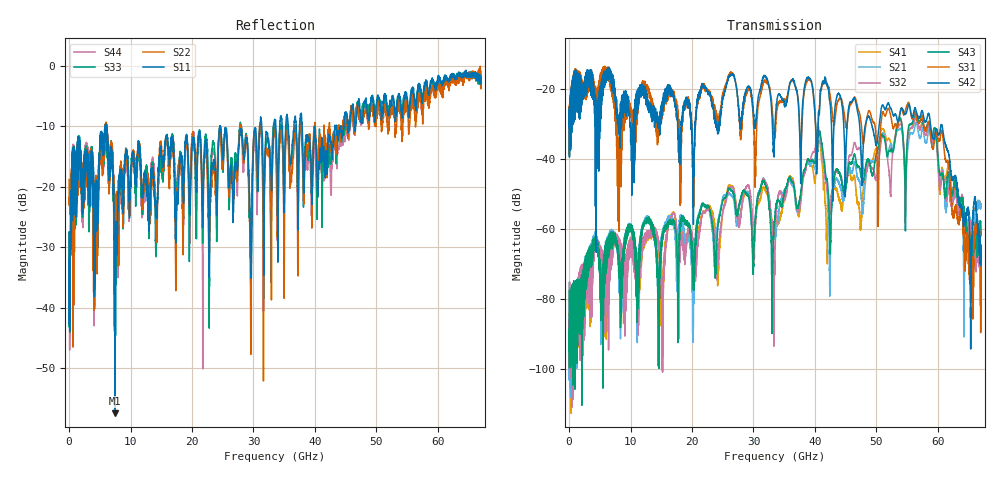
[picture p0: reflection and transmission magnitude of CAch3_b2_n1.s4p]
!Agilent Technologies,N5247A,US51170199,A.09.90.13
!Agilent N5247A: A.09.90.13
!Date: Wednesday, October 17, 2018 17:19:54
!Correction: S11(Full 4 Port(1,2,3,4))
!S12(Full 4 Port(1,2,3,4))
!S13(Full 4 Port(1,2,3,4))
!S14(Full 4 Port(1,2,3,4))
!S21(Full 4 Port(1,2,3,4))
!S22(Full 4 Port(1,2,3,4))
!S23(Full 4 Port(1,2,3,4))
!S24(Full 4 Port(1,2,3,4))
!S31(Full 4 Port(1,2,3,4))
!S32(Full 4 Port(1,2,3,4))
!S33(Full 4 Port(1,2,3,4))
!S34(Full 4 Port(1,2,3,4))
!S41(Full 4 Port(1,2,3,4))
!S42(Full 4 Port(1,2,3,4))
!S43(Full 4 Port(1,2,3,4))
!S44(Full 4 Port(1,2,3,4))
!S4P File: Measurements: <S11,S12,S13,S14>,
!<S21,S22,S23,S24>,
!<S31,S32,S33,S34>,
!<S41,S42,S43,S44>:
# Hz S  dB  R 50
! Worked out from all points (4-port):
!   6701 points, 10 MHz to 67 GHz, reference 50 ohm
!   strongest paths, dB at 10 MHz, 16.76 GHz, 33.51 GHz, 50.25 GHz, 67 GHz:
!     S42: -31.1, -20.4, -30.1, -33.6, -68.2
!     S31: -30.3, -21.1, -33.2, -50.9, -83.5
!     S43: -90.9, -57.6, -56.7, -37.1, -57.9
!     S32: -98.4, -56.1, -64.7, -42.6, -75.1
!     S21: -93.8, -56.8, -68.0, -39.7, -53.5
!     S41: -84.3, -55.7, -61.0, -37.0, -53.4
!   lowest |S11| = -57.5 dB at 7.449 GHz (marker M1), VSWR 1.00, Z = 49.9 - j0.107 ohm
!   |S11| at or under -10 dB: start of sweep to 5.92 GHz; 6.065 GHz to 24.53 GHz (18.47 GHz wide, 121 % of centre); 24.62 GHz to 31.03 GHz (6.411 GHz wide, 23 % of centre)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
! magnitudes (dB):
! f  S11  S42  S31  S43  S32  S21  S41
! 10 MHz  -27.5  -31.1  -30.3  -90.9  -98.4  -93.8  -84.3
! 7.449 GHz  -57.5  -19.9  -22.2  -61.3  -61.0  -61.0  -61.6
! 33.35 GHz  -9.4  -39.3  -32.8  -59.6  -77.1  -73.8  -60.3
! 40.52 GHz  -18.1  -29.6  -30.1  -32.6  -30.6  -33.8  -36.3
! 42.41 GHz  -11.7  -23.6  -21.0  -60.0  -54.5  -71.5  -54.0
! 56.44 GHz  -7.0  -26.1  -27.5  -27.1  -27.8  -29.6  -28.1
! 67 GHz  -2.9  -68.2  -83.5  -57.9  -75.1  -53.5  -53.4
